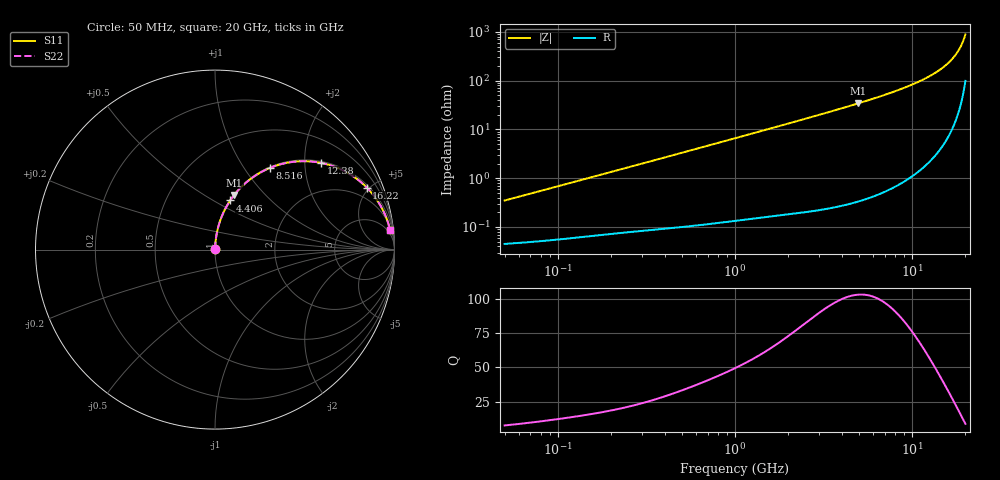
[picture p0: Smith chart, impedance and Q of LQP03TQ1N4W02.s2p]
!Murata Part Number: LQP03TQ1N4W02
!These Parameters are Measured in Series Mode Connection
!  o--[Z]--o
!Port1  Port2
!  o-------o
!Freq. Start=50[MHz] Stop=20[GHz], 401[Steps]
# Hz S RI R 50
!Freq.(Hz) S11(Real) S11(Imag) S21(Real) S21(Imag) S12(Real) S12(Imag) S22(Real) S22(Imag)
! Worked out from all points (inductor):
!   401 points, 50 MHz to 20 GHz, reference 50 ohm
!   read as one part in series: L = 1.1 nH near 51.52 MHz
!   highest Q = 103 at 4.967 GHz (marker M1), where L = 1.1 nH
!   S11 on the Smith chart (normalised r, x): 50 MHz: 1.00, +0.01; 4.406 GHz: 1.01, +0.60; 8.516 GHz: 1.02, +1.32; 12.38 GHz: 1.04, +2.40; 16.22 GHz: 1.15, +4.82; 20 GHz: 3, +18
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5e7  0.000463 0.00346  0.9995 -0.00346  0.9995 -0.00346  0.000463 0.00346
1.364002e8  0.000708 0.00924  0.9993 -0.00924  0.9993 -0.00924  0.000708 0.00924
3.721004e8  0.00151 0.0247  0.9985 -0.0247  0.9985 -0.0247  0.00151 0.0247
1e9  0.00565 0.0655  0.9944 -0.0655  0.9944 -0.0655  0.00565 0.0655
1.714689e9  0.0143 0.1113  0.9857 -0.1113  0.9857 -0.1113  0.0143 0.1113
2.728004e9  0.0337 0.1748  0.9663 -0.1748  0.9663 -0.1748  0.0337 0.1748
4.405649e9  0.085 0.274  0.915 -0.274  0.915 -0.274  0.085 0.274
4.966507e9  0.1073 0.3047  0.8927 -0.3047  0.8927 -0.3047  0.1073 0.3047
6.125241e9  0.1615 0.3631  0.8385 -0.3631  0.8385 -0.3631  0.1615 0.3631
7.442007e9  0.2353 0.4189  0.7647 -0.4189  0.7647 -0.4189  0.2353 0.4189
8.516016e9  0.3041 0.4543  0.6959 -0.4543  0.6959 -0.4543  0.3041 0.4543
1.050288e10  0.4465 0.4902  0.5535 -0.4902  0.5535 -0.4902  0.4465 0.4902
1.238412e10  0.5893 0.4834  0.4107 -0.4834  0.4107 -0.4834  0.5893 0.4834
1.334722e10  0.6609 0.4637  0.3391 -0.4637  0.3391 -0.4637  0.6609 0.4637
1.438523e10  0.7339 0.4306  0.2661 -0.4306  0.2661 -0.4306  0.7339 0.4306
1.527346e10  0.7912 0.3933  0.2088 -0.3933  0.2088 -0.3933  0.7912 0.3933
1.621653e10  0.8453 0.346  0.1547 -0.346  0.1547 -0.346  0.8453 0.346
1.721783e10  0.8939 0.2886  0.1061 -0.2886  0.1061 -0.2886  0.8939 0.2886
1.800918e10  0.9253 0.2394  0.0747 -0.2394  0.0747 -0.2394  0.9253 0.2394
1.88369e10  0.9511 0.1856  0.0489 -0.1856  0.0489 -0.1856  0.9511 0.1856
1.940974e10  0.9648 0.1476  0.0352 -0.1476  0.0352 -0.1476  0.9648 0.1476
2e10  0.9754 0.1083  0.0246 -0.1083  0.0246 -0.1083  0.9754 0.1083
